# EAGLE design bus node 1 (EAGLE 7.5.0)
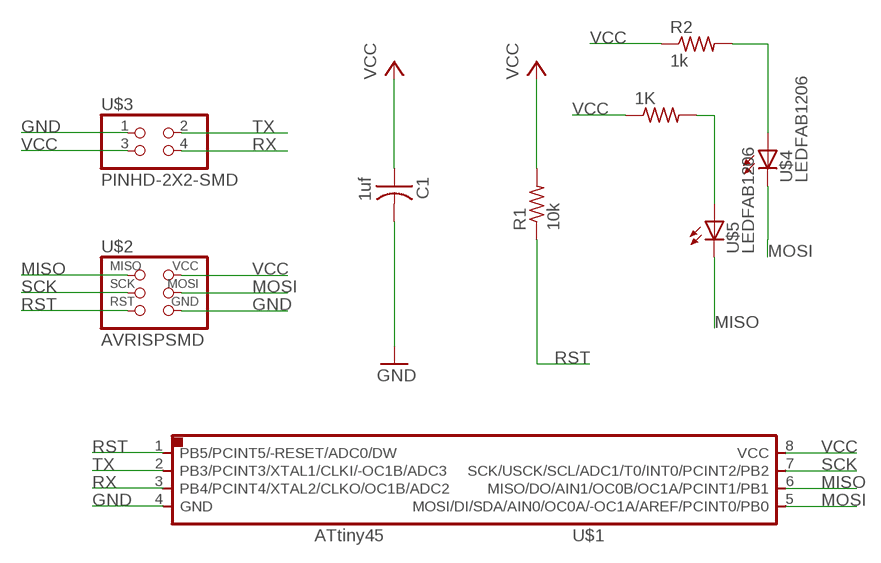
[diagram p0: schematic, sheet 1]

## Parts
1K  RES-US1206FAB  [R1206FAB]
C1  1uf  CAP-US1206FAB  [C1206FAB]
R1  10k  RES-US1206FAB  [R1206FAB]
R2  1k  RES-US1206FAB  [R1206FAB]
U$1  ATTINY45SI  [SOIC8]
U$2  AVRISPSMD  [2X03SMD]
U$3  PINHD-2X2-SMD  [2X02SMD]
U$4  LEDFAB1206  [LED1206FAB]
U$5  LEDFAB1206  [LED1206FAB]

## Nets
GND: C1.2 U$1.4(GND) U$2.6(GND) U$3.1
MISO: U$1.6(MISO/DO/AIN1/OC0B/OC1A/PCINT1/PB1) U$2.1(MISO) U$5.2(C)
MOSI: U$1.5(MOSI/DI/SDA/AIN0/OC0A/-OC1A/AREF/PCINT0/PB0) U$2.4(MOSI) U$4.2(C)
N$2: R2.2 U$4.1(A)
N$3: 1K.2 U$5.1(A)
RST: R1.1 U$1.1(PB5/PCINT5/-RESET/ADC0/DW) U$2.5(RST)
RX: U$1.3(PB4/PCINT4/XTAL2/CLKO/OC1B/ADC2) U$3.4
SCK: U$1.7(SCK/USCK/SCL/ADC1/T0/INT0/PCINT2/PB2) U$2.3(SCK)
TX: U$1.2(PB3/PCINT3/XTAL1/CLKI/-OC1B/ADC3) U$3.2
VCC: 1K.1 C1.1 R1.2 R2.1 U$1.8(VCC) U$2.2(VCC) U$3.3

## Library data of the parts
1K R1 R2 = fab:RES-US: Resistor (US Symbol)
C1 = fab:CAP-US
U$1 = fab:ATTINY45
U$2 = fab:AVRISP
U$3 = fab:PINHD-2X2-SMD
U$4 U$5 = fab:LED: LED

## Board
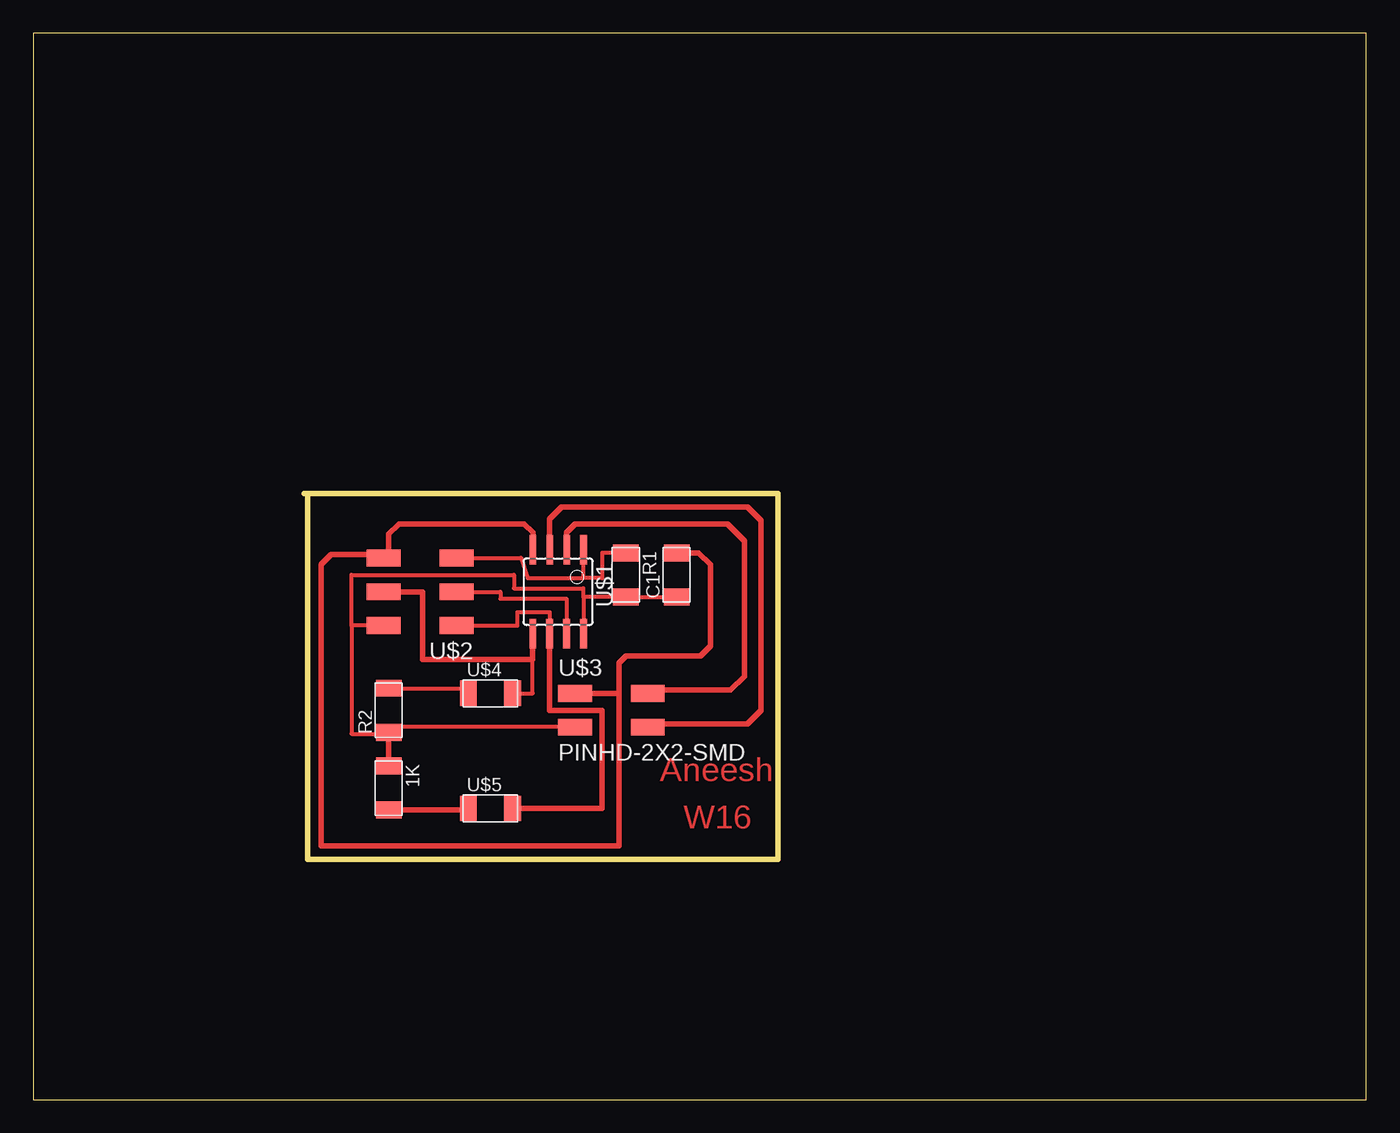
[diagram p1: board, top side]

Size 100 x 80 mm. Coordinates in mm from the lower left corner, seen from the top.
Outline: 20.32,45.47 20.57,45.47
Outline: 20.57,45.47 55.88,45.47 55.88,18.03 20.57,18.03 20.57,45.47
Outline: 0,0 100,0 100,80 0,80 0,0
Copper layers (1*16): Top 0.035mm / dielectric 1.5mm / Bottom 0.035mm
Design rules "default": minimum track width 10mil, minimum drill 24mil, track to track 8mil, track to pad 8mil, pad to pad 8mil, via to via 8mil, smd to smd 8mil, copper to edge 40mil, drill to drill 8mil, minimum pad ring 10mil, minimum via ring 8mil, stop-mask expansion 4mil, vias tented up to drill 0mil, thermal gap 10mil

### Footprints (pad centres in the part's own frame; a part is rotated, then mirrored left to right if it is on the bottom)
R1206FAB = smd 1.27 x 1.905: 1 -1.651,0; 2 1.651,0
C1206FAB = smd 1.27 x 1.905: 1 -1.651,0; 2 1.651,0
SOIC8 = smd 0.5 x 2.2: 1 -1.905,-3.154; 2 -0.645,-3.154; 3 0.625,-3.154; 4 1.895,-3.154; 5 1.905,3.154; 6 0.635,3.154; 7 -0.635,3.154; 8 -1.905,3.154
2X03SMD = smd 2.54 x 1.27: 1 -2.54,2.54; 2 2.92,2.54; 3 -2.54,0; 4 2.92,0; 5 -2.54,-2.54; 6 2.92,-2.54
2X02SMD = smd 2.54 x 1.27: 1 -2.54,1.27; 2 2.92,1.27; 3 -2.54,-1.27; 4 2.92,-1.27
LED1206FAB = smd 1.27 x 1.905: 1 -1.651,0; 2 1.651,0

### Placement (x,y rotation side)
1K  26.67,23.37 270 top
C1  48.26,39.37 90 top
R1  44.45,39.37 270 top
R2  26.67,29.21 90 top
U$1  39.37,38.1 180 top
U$2  29.21,38.1 180 top
U$3  43.18,29.21 0 top
U$4  34.29,30.48 0 top
U$5  34.29,21.84 0 top

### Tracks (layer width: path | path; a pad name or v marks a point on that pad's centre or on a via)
GND
  Top 0.406: C1.2 49.91,41.02 50.8,40.13 50.8,34.04 50.04,33.27 44.45,33.27 43.94,32.77 43.94,30.48 | U$1.4 37.48,42.53 36.83,43.18 27.43,43.18 26.67,42.42 26.67,40.64 U$2.6 26.04,40.89 22.35,40.89 21.59,40.13 21.59,19.05 43.94,19.05 43.94,30.48 | U$3.1 43.94,30.48
MISO
  Top 0.305: U$2.1 36.32,35.56 36.32,36.58 38.73,36.58 U$1.6
  Top 0.406: U$5.2 42.67,21.84 42.67,29.21 38.73,29.21 U$1.6
MOSI
  Top 0.305: U$4.2 37.47,30.48 37.47,33.02
  Top 0.406: U$2.4 29.21,38.1 29.21,33.02 37.47,33.02 U$1.5
N$2
  Top 0.305: R2.2 32.64,30.86 U$4.1
N$3
  Top 0.406: 1K.2 32.64,21.72 U$5.1
RST
  Top 0.305: U$2.5 36.58,40.64 37.08,39.12 41.27,39.12 | 41.27,39.12 U$1.1 | R1.1 42.67,41.02 42.67,39.12 41.27,39.12
RX
  Top 0.406: U$3.4 46.35,28.19 53.59,28.19 54.61,29.21 54.61,43.43 53.59,44.45 39.62,44.45 38.74,43.57 U$1.3
SCK
  Top 0.305: U$2.3 35.05,38.1 35.05,37.59 40.01,37.59 U$1.7
TX
  Top 0.406: U$3.2 46.35,30.73 52.32,30.73 53.34,31.75 53.34,41.91 52.07,43.18 40.64,43.18 40.02,42.55 U$1.2
VCC
  Top 0.305: 23.88,35.56 23.88,39.37 36.07,39.37 36.07,38.35 41.27,38.35 41.27,37.72 | 41.27,37.72 U$1.8 | 41.27,37.72 R1.2 C1.1 | U$2.2 23.88,35.56 | 23.88,35.56 23.88,27.43 26.67,27.43 R2.1 26.67,27.94 U$3.3
  Top 0.406: 1K.1 R2.1

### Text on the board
Top: Aneesh | W16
